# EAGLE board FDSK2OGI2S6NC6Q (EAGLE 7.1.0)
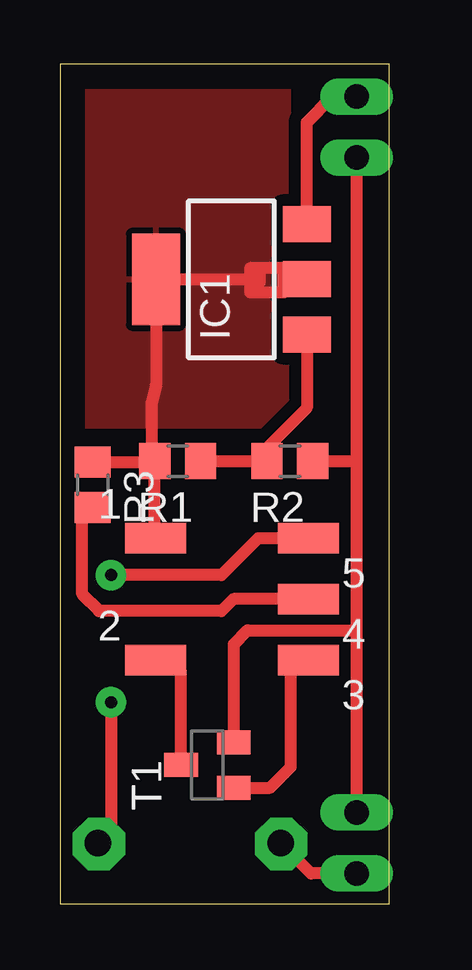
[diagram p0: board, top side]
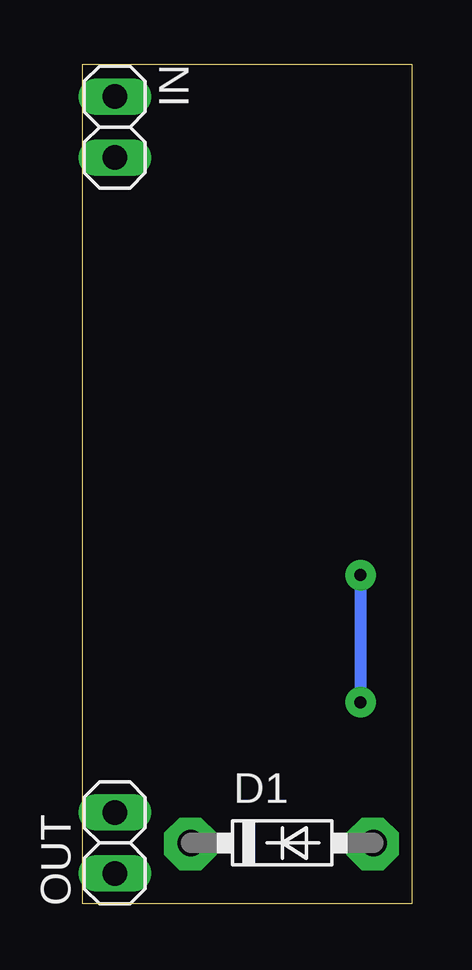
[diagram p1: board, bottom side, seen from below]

Size 13.73 x 35 mm. Coordinates in mm from the lower left corner, seen from the top.
Outline: 0,0 13.73,0 13.73,35 0,35 0,0
Copper layers (1*16): Top 0.035mm / dielectric 1.5mm / Bottom 0.035mm
Design rules "default": minimum track width 10mil, minimum drill 24mil, track to track 8mil, track to pad 8mil, pad to pad 8mil, via to via 8mil, smd to smd 8mil, copper to edge 40mil, drill to drill 8mil, minimum pad ring 10mil, minimum via ring 8mil, stop-mask expansion 4mil, vias tented up to drill 0mil, thermal gap 10mil

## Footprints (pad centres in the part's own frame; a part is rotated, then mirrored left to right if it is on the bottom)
SMD1,27-2,54 = smd 1.27 x 2.54: 1 0,0
DO41-7.6 = drill 1.1 pad 1.7: A 3.81,0; C -3.81,0
SOT223 = smd 1.5 x 2: 1 -2.3,-3.15; 2 0,-3.15; 3 2.3,-3.15 | smd 3.8 x 2: 4 0,3.15
1X02 = drill 1.016 long: 1 -1.27,0; 2 1.27,0
R0805 = smd 1.3 x 1.5: 1 -0.95,0; 2 0.95,0
SOT23 = smd 1 x 1.4: 1 -0.95,-1.1; 2 0.95,-1.1; 3 0,1.1

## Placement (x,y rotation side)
1  [SMD1,27-2,54]  3.98,15.24 270 top
2  [SMD1,27-2,54]  3.98,10.16 270 top
3  [SMD1,27-2,54]  10.36,10.16 90 top
4  [SMD1,27-2,54]  10.36,12.7 90 top
5  [SMD1,27-2,54]  10.36,15.24 90 top
D1  1N5817-B  [DO41-7.6]  5.4,2.54 0 bottom
IC1  LM317MBSTT3  [SOT223]  7.15,26.04 90 top
IN  [1X02]  12.38,32.38 270 bottom
OUT  [1X02]  12.38,2.54 90 bottom
R1  270  [R0805]  4.91,18.45 180 top
R2  56  [R0805]  9.59,18.45 180 top
R3  1k  [R0805]  1.37,17.47 270 top
T1  BC846  [SOT23]  6.15,5.79 90 top

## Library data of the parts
1-5 = wirepad
D1 = diode
IC1 = v-reg
IN OUT = pinhead
R1-R3 = rcl
T1 = transistor

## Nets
+5V: IC1.3 IN.1
GND: IN.2 OUT.2 R2.1 T1.2
N$1: 1.1 IC1.4 R1.2 R3.1
N$2: IC1.1 R1.1 R2.2
N$3: 5.1 D1.A
N$4: 3.1 T1.1
N$5: 2.1 T1.3
N$6: 4.1 R3.2
N$7: D1.C OUT.1

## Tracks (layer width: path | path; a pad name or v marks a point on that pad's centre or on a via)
+5V
  Top 0.5: IC1.3 10.3,32.57 11.33,33.6 12.33,33.6 IN.1
GND
  Top 0.5: OUT.2 12.38,11.4 | 12.38,11.4 12.38,18.5 | 12.38,18.5 IN.2 | T1.2 7.25,10.82 7.83,11.4 12.38,11.4 | R2.1 12.33,18.45 12.38,18.5
N$1
  Top 0.5: 8.33,26.5 9.33,26.5 9.33,25.5 7.93,25.5 7.93,26.5 8.33,26.5 | 8.33,26.5 8.33,26 | 8.33,26 8.33,25.9 | 8.33,26 8.29,26.04 IC1.4 4,21.63 3.83,20.9 3.83,18.58 R1.2 3.93,18.42 | R3.1 3.93,18.42 | 3.93,18.42 3.93,15.89 1.1
  pour Top (isolate 0.5): 0.63,34.4 9.53,34.4 9.53,19.9 0.63,19.9
N$2
  Top 0.5: R1.1 R2.2 8.73,18.54 8.73,19.1 10.3,20.67 IC1.1
N$3  (via drill 0.5 pad 1.27, 0.8 pad 2.18)
  Top 0.5: 5.1 8.27,15.24 6.73,13.7 v2.13,13.7 | v2.13,8.4 2.13,3.18 D1.A v1.63,2.5
  Bottom 0.5: v2.13,13.7 v2.13,8.4
N$4
  Top 0.5: T1.1 8.77,4.84 9.63,5.7 9.63,10.13 3.1
N$5
  Top 0.5: T1.3 5.05,9.69 2.1
N$6
  Top 0.5: 4.1 7.23,12.7 6.73,12.2 1.63,12.2 0.93,12.9 0.93,16.18 R3.2
N$7  (via drill 0.8 pad 2.18)
  Top 0.5: OUT.1 10.48,1.27 D1.C 9.21,2.52 v9.23,2.5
